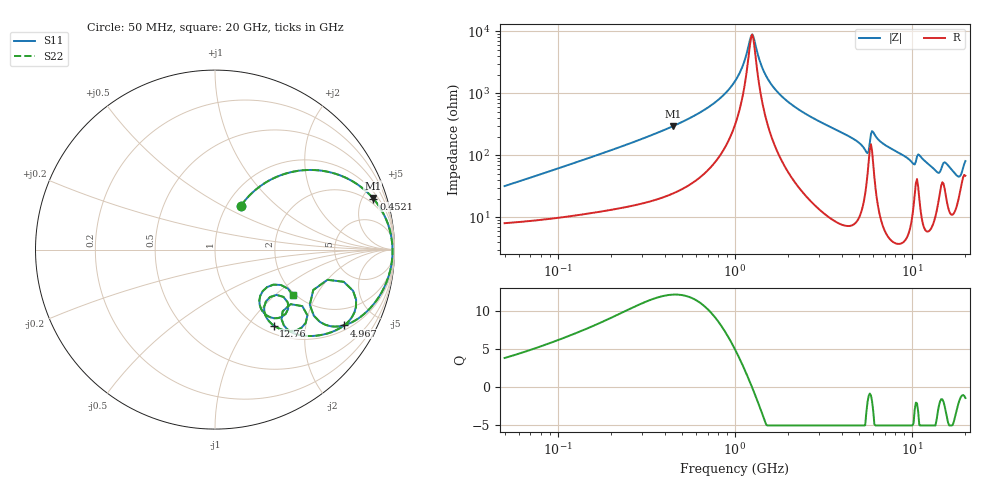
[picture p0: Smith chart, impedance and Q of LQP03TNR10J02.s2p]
!Murata Part Number: LQP03TNR10J02
!These Parameters are Measured in Series Mode Connection
!  o--[Z]--o
!Port1  Port2
!  o-------o
!Freq. Start=50[MHz] Stop=20[GHz], 401[Steps]
# Hz S RI R 50
!Freq.(Hz) S11(Real) S11(Imag) S21(Real) S21(Imag) S12(Real) S12(Imag) S22(Real) S22(Imag)
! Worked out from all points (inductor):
!   401 points, 50 MHz to 20 GHz, reference 50 ohm
!   read as one part in series: L = 97.8 nH near 51.52 MHz
!   highest Q = 12.1 at 445.4 MHz (marker M1), where L = 105 nH
!   self-resonance near 1.233 GHz
!   S11 on the Smith chart (normalised r, x): 50 MHz: 1.16, +0.62; 452.1 MHz: 1.49, +6.01; 4.967 GHz: 1.19, -3.27; 12.76 GHz: 1.13, -1.34; 20 GHz: 1.94, -1.32
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5e7  0.1453 0.2454  0.8547 -0.2454  0.8547 -0.2454  0.1453 0.2454
1.364002e8  0.4198 0.4306  0.5802 -0.4306  0.5802 -0.4306  0.4198 0.4306
3.721004e8  0.8295 0.3362  0.1705 -0.3362  0.1705 -0.3362  0.8295 0.3362
4.45371e8  0.8785 0.2881  0.1215 -0.2881  0.1215 -0.2881  0.8785 0.2881
4.520922e8  0.8821 0.284  0.1179 -0.284  0.1179 -0.284  0.8821 0.284
7.411344e8  0.9632 0.1435  0.0368 -0.1435  0.0368 -0.1435  0.9632 0.1435
1e9  0.9839 0.0605  0.0161 -0.0605  0.0161 -0.0605  0.9839 0.0605
1.251922e9  0.9889 -0.00073  0.0111 0.00073  0.0111 0.00073  0.9889 -0.00073
1.432596e9  0.988 -0.0376  0.012 0.0376  0.012 0.0376  0.988 -0.0376
1.639343e9  0.9841 -0.0751  0.0159 0.0751  0.0159 0.0751  0.9841 -0.0751
2.728004e9  0.9347 -0.2267  0.0653 0.2267  0.0653 0.2267  0.9347 -0.2267
4.966507e9  0.7171 -0.4226  0.2829 0.4226  0.2829 0.4226  0.7171 -0.4226
5.515528e9  0.5506 -0.3685  0.4494 0.3685  0.4494 0.3685  0.5506 -0.3685
5.856089e9  0.7171 -0.1794  0.2829 0.1794  0.2829 0.1794  0.7171 -0.1794
6.125241e9  0.7853 -0.3202  0.2147 0.3202  0.2147 0.3202  0.7853 -0.3202
7.442007e9  0.6371 -0.464  0.3629 0.464  0.3629 0.464  0.6371 -0.464
1.050288e10  0.4213 -0.304  0.5787 0.304  0.5787 0.304  0.4213 -0.304
1.276073e10  0.3271 -0.4229  0.6729 0.4229  0.6729 0.4229  0.3271 -0.4229
1.417136e10  0.2834 -0.2898  0.7166 0.2898  0.7166 0.2898  0.2834 -0.2898
1.527346e10  0.4079 -0.3297  0.5921 0.3297  0.5921 0.3297  0.4079 -0.3297
1.800918e10  0.2471 -0.2823  0.7529 0.2823  0.7529 0.2823  0.2471 -0.2823
2e10  0.434 -0.2538  0.566 0.2538  0.566 0.2538  0.434 -0.2538
